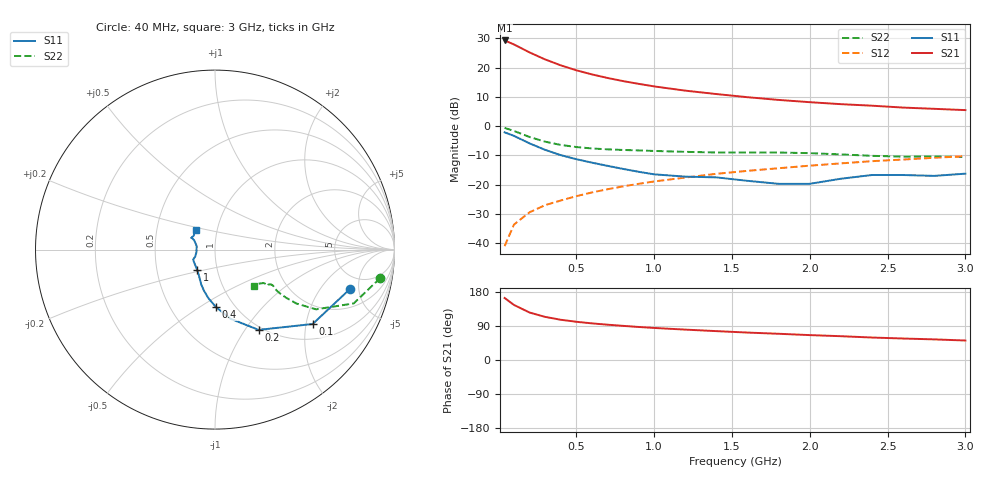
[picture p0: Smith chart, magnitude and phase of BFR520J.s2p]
! Filename:  BFR520J.S2P  Version:  2.1
! Philips part #: BFR520  Date: Sep 1991
! Bias condition: Vce=6V, Ic=15mA
#  MHz  S  MA  R  50
! Freq  S11  S21  S12  S22  !GUM [dB]
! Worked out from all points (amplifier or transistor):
!   21 points, 40 MHz to 3 GHz, reference 50 ohm
!   highest |S21| = 29.2 dB at 40 MHz (marker M1)
!   |S21| within 3 dB of that: start of sweep to 160.7 MHz
!   unconditionally stable (mu >= 1): 1.008 GHz to end of sweep
!   at 300 MHz: K = 0.71, MSG = 24.8 dB, |S12| = -26.9 dB
!   at 1 GHz: K = 1.00, MSG = 16.2 dB, |S12| = -18.9 dB
!   at 3 GHz: K = 1.02, MAG = 7.1 dB, |S12| = -10.2 dB
!   lowest NFmin = 1.30 dB at 500 MHz
!   S11 on the Smith chart (normalised r, x): 40 MHz: 3.54, -4.02; 100 MHz: 1.40, -2.18; 200 MHz: 0.96, -1.16; 400 MHz: 0.82, -0.59; 1 GHz: 0.80, -0.19; 3 GHz: 0.79, +0.18
40  0.784 -16.2  28.91 163.7  0.009 83.1  0.934 -9.8
100  0.684 -37.3  24.73 145.3  0.021 73.3  0.829 -21.2
200  0.509 -61.5  18.11 125.3  0.034 67.4  0.654 -30.6
300  0.395 -77.3  13.73 113.8  0.045 67.2  0.544 -33.5
400  0.321 -88.9  10.9 106.2  0.054 67.8  0.479 -34.1
500  0.274 -97.6  8.977 100.9  0.064 68.9  0.441 -34.0
600  0.239 -104.6  7.637 96.7  0.074 69.6  0.417 -33.7
700  0.211 -111.0  6.644 93.2  0.084 70.8  0.403 -33.2
800  0.187 -116.7  5.871 90.1  0.094 71.4  0.393 -32.5
900  0.167 -122.9  5.269 87.2  0.104 71.7  0.386 -32.1
1000  0.151 -131.0  4.765 84.6  0.114 71.9  0.378 -31.8
1200  0.138 -145.4  4.034 80.2  0.133 71.8  0.365 -31.9
1400  0.134 -155.5  3.528 76.2  0.154 71.3  0.356 -33.2
1600  0.117 -160.6  3.118 72.4  0.173 70.7  0.355 -33.5
1800  0.104 -172.5  2.802 69.2  0.192 70.3  0.355 -34.4
2000  0.104 168.9  2.564 65.7  0.212 69.2  0.347 -34.1
2200  0.127 155.9  2.372 62.8  0.232 68.2  0.33 -34.4
2400  0.147 152.9  2.234 59.3  0.253 66.9  0.312 -37.2
2600  0.147 154.1  2.074 56.7  0.27 65.6  0.302 -40.9
2800  0.142 146.9  1.975 54.4  0.289 64.9  0.304 -42.9
3000  0.155 133.8  1.878 51.4  0.308 63.6  0.298 -42.4
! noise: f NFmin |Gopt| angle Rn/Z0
500  1.3  0.25  25  0.24
900  1.45  0.218  45  0.25
1000  1.5  0.205  53  0.28
2000  2.05  0.135  167  0.17
